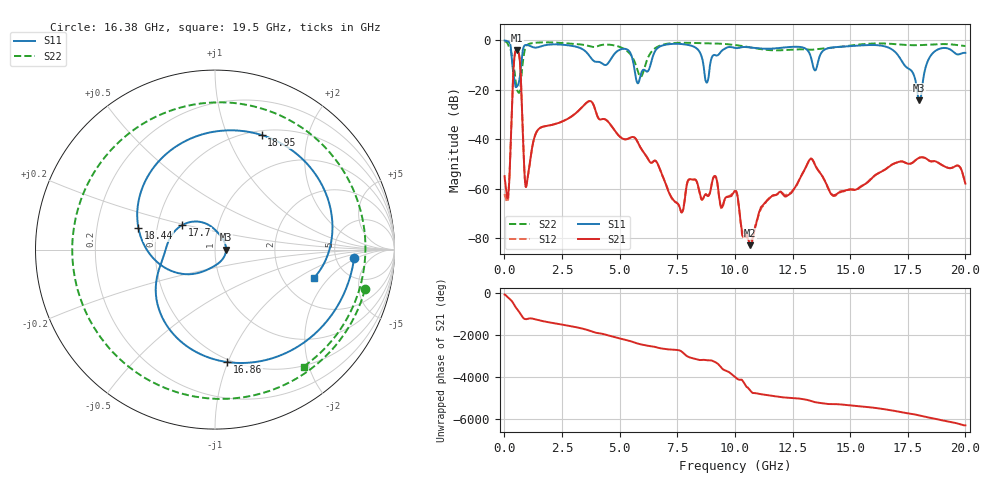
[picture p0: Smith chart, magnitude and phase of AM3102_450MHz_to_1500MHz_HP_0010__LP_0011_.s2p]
!Agilent Technologies,E8364B,MY43040894,A.07.50.67
!Agilent E8364B: A.07.50.67
!Date: Thursday, January 11, 2018 05:24:24
!Correction: S11(Full 2 Port(1,2))
!S21(Full 2 Port(1,2))
!S12(Full 2 Port(1,2))
!S22(Full 2 Port(1,2))
!S2P File: Measurements: S11, S21, S12, S22:
# Hz S  dB  R 50
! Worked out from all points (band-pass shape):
!   1601 points, 10 MHz to 20 GHz, reference 50 ohm
!   highest |S21| = -3.89 dB at 534.7 MHz (marker M1); lowest = -82.9 dB at 10.67 GHz (marker M2)
!   |S21| within 3 dB of the highest: 435.6 MHz to 655.7 MHz (220.1 MHz wide, 40.3 % of centre)
!   lowest |S11| = -24.2 dB at 18 GHz (marker M3), VSWR 1.13, Z = 56.6 + j0.0298 ohm
!   |S11| at or under -10 dB: 348.3 MHz to 726.8 MHz (378.5 MHz wide, 70.4 % of centre); 5.612 GHz to 6.337 GHz (725.7 MHz wide, 12.1 % of centre); 17.35 GHz to 18.3 GHz (951.4 MHz wide, 5.34 % of centre)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
!   |S22| runs from -21.3 to -0.4 dB; largest |S21 - S12| = 0.002
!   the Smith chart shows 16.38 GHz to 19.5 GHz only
!   S11 on the Smith chart (normalised r, x): 16.38 GHz: 7.48, -1.84; 16.86 GHz: 0.48, -0.99; 17.7 GHz: 0.67, +0.19; 18.44 GHz: 0.39, +0.12; 18.95 GHz: 0.55, +1.34; 19.5 GHz: 2.98, -1.39
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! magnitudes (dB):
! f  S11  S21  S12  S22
! 10 MHz  -0.1  -54.9  -62.2  -0.4
! 184.9 MHz  -0.6  -60.8  -61.3  -2.4
! 534.7 MHz  -18.7  -3.9  -3.9  -19.6
! 959.5 MHz  -1.9  -58.6  -58.6  -2.2
! 1.459 GHz  -2.8  -36.2  -36.2  -0.9
! 3.346 GHz  -3.4  -27.3  -27.3  -1.7
! 5.795 GHz  -17.4  -41.4  -41.4  -12.6
! 6.682 GHz  -2.9  -50.6  -50.6  -2.4
! 7.669 GHz  -1.5  -69.5  -69.4  -1.0
! 8.781 GHz  -17.1  -62.7  -62.6  -1.2
! 10.01 GHz  -3.1  -61.1  -60.9  -1.9
! 10.67 GHz  -2.9  -82.9  -83.2  -2.9
! 13.34 GHz  -8.4  -48.1  -48.0  -3.8
! 16.38 GHz  -2.2  -53.0  -52.9  -1.3
! 16.68 GHz  -3.0  -51.2  -51.1  -1.4
! 16.86 GHz  -4.0  -50.0  -50.1  -1.5
! 17.7 GHz  -12.9  -49.6  -49.5  -2.0
! 18 GHz  -24.2  -47.5  -47.5  -2.0
! 18.44 GHz  -7.1  -48.8  -48.8  -1.8
! 18.95 GHz  -3.2  -50.2  -50.3  -1.5
! 19.5 GHz  -4.8  -51.3  -51.1  -1.8
! 20 GHz  -5.1  -58.0  -57.3  -2.3
